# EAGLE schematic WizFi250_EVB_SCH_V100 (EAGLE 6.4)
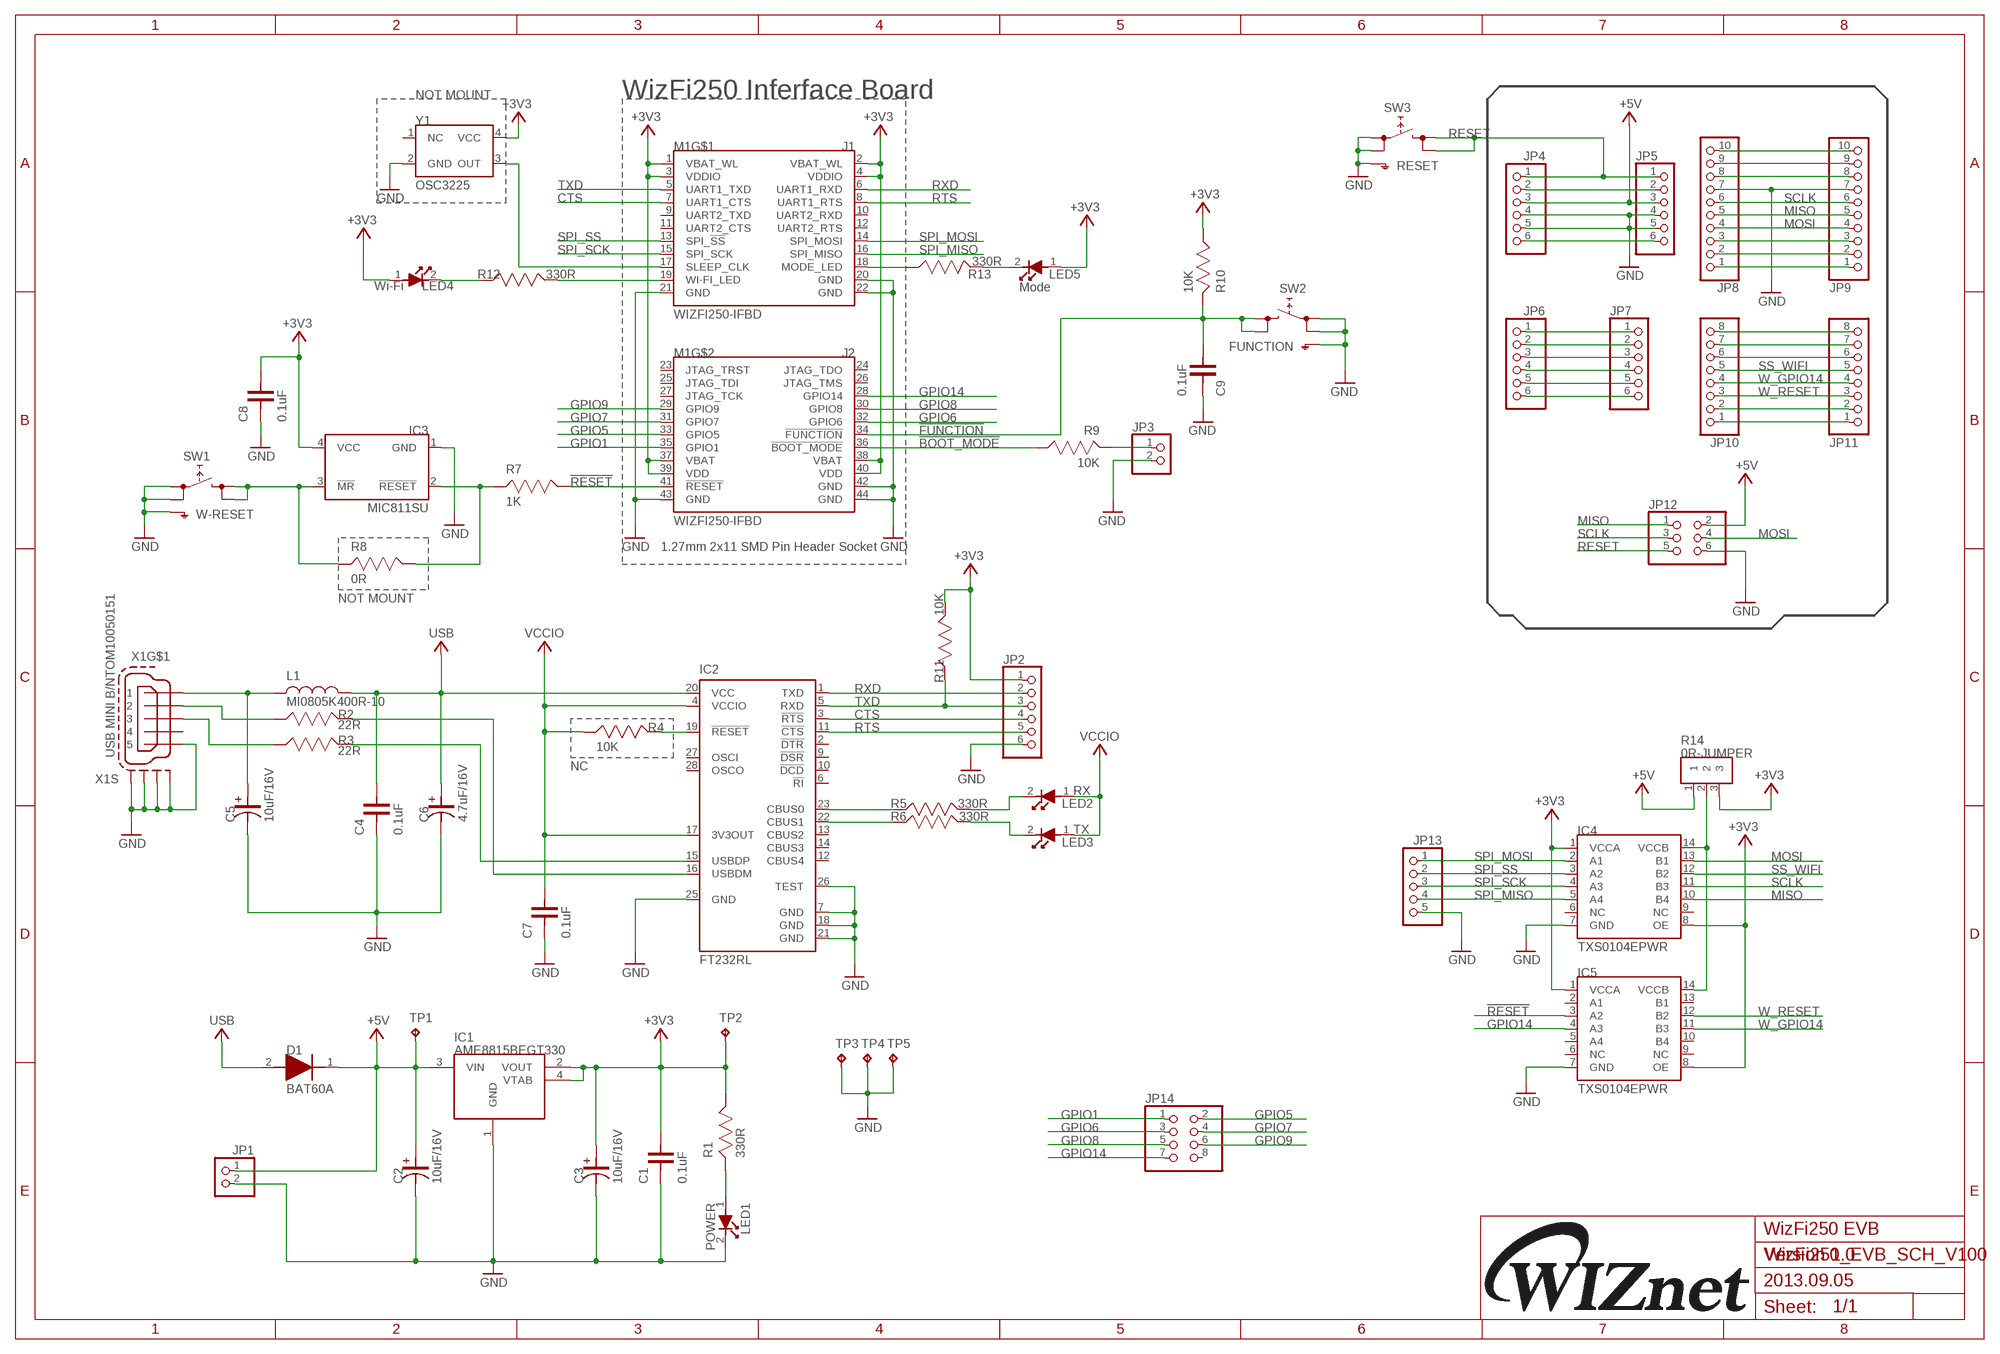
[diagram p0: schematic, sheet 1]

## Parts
C1  0.1uF  C-1608  [C-1608]
C2  10uF/16V  C-3216(TANTAL)  [C-3216(TANTAL)]
C3  10uF/16V  C-3216(TANTAL)  [C-3216(TANTAL)]
C4  0.1uF  C-1608  [C-1608]
C5  10uF/16V  C-3216(TANTAL)  [C-3216(TANTAL)]
C6  4.7uF/16V  C-3216(TANTAL)  [C-3216(TANTAL)]
C7  0.1uF  C-1608  [C-1608]
C8  0.1uF  C-1608  [C-1608]
C9  0.1uF  C-1608  [C-1608]
D1  BAT60A  [BAT60A]
IC1  AME8815BEGT330  [SOT-223]
IC2  FT232RL  [SSOP28]
IC3  MIC811SU  [MIC811SU]
IC4  TXS0104EPWR  [TXS0104EPWR]
IC5  TXS0104EPWR  [TXS0104EPWR]
JP1  PINHD-1X2  [1X02]
JP2  PINHD-1X6  [1X06]
JP3  PINHD-1X2  [1X02]
JP4  PINHD-1X6  [1X06]
JP5  PINHD-1X6  [1X06]
JP6  PINHD-1X6  [1X06]
JP7  PINHD-1X6  [1X06]
JP8  PINHD-1X10  [1X10]
JP9  PINHD-1X10  [1X10]
JP10  PINHD-1X8  [1X08]
JP11  PINHD-1X8  [1X08]
JP12  PINHD-2X3  [2X03]
JP13  PINHD-1X5  [1X05]
JP14  PINHD-2X4  [2X04]
L1  MI0805K400R-10  L-2012  [L-2012]
LED1  POWER  LED-1608  [LED-1608]
LED2  RX  LED-1608  [LED-1608]
LED3  TX  LED-1608  [LED-1608]
LED4  Wi-Fi  LED-1608  [LED-1608]
LED5  Mode  LED-1608  [LED-1608]
M1  WIZFI250-IFBD  [WIZFI250-IFBD]
R1  330R  R-1608  [R-1608]
R2  22R  R-1608  [R-1608]
R3  22R  R-1608  [R-1608]
R4  10K  R-1608  [R-1608]
R5  330R  R-1608  [R-1608]
R6  330R  R-1608  [R-1608]
R7  1K  R-1608  [R-1608]
R8  0R  R-1608  [R-1608]
R9  10K  R-1608  [R-1608]
R10  10K  R-1608  [R-1608]
R11  10K  R-1608  [R-1608]
R12  330R  R-1608  [R-1608]
R13  330R  R-1608  [R-1608]
R14  0R-JUMPER  R-1608-JUMPER  [R-1608-JUMPER]
SW1  W-RESET  SKHMPSE010  [SKHMPXE010]
SW2  FUNCTION  SKHMPSE010  [SKHMPXE010]
SW3  RESET  SKHMPSE010  [SKHMPXE010]
TP1  TPB1,27  [B1,27]
TP2  TPB1,27  [B1,27]
TP3  TPB1,27  [B1,27]
TP4  TPB1,27  [B1,27]
TP5  TPB1,27  [B1,27]
X1  USB MINI B/NTOM10050151  MINI-USB-SCHIELD-32005-201  [32005-201]
Y1  OSC3225  [OSC3225]

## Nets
!BOOT_MODE: M1.36(!BOOT_MODE) R9.2
!FUNCTION: C9.2 M1.34(!FUNCTION) R10.1 SW2.3(2.1) SW2.4(2.2)
!RESET: IC5.3(A2) M1.41(!RESET) R7.2
+3V3: C1.2 C3.1 C8.2 IC1.2(VOUT) IC1.4(VTAB) IC3.4(VCC) IC4.1(VCCA) IC4.8(OE) IC5.1(VCCA) IC5.8(OE) JP2.1 LED4.1 LED5.1 M1.1(VBAT_WL) M1.2(VBAT_WL) M1.3(VDDIO) M1.4(VDDIO) M1.37(VBAT) M1.38(VBAT) M1.39(VDD) M1.40(VDD) R1.2 R10.2 R11.2 R14.3 TP2.TP Y1.4(VCC)
+5V: C2.1 D1.1 IC1.3(VIN) JP1.1 JP4.3 JP5.3 JP12.2 R14.1 TP1.TP
CTS: IC2.3(!RTS) JP2.4 M1.7(UART1_CTS)
GND: C1.1 C2.2 C3.2 C4.1 C5.2 C6.2 C7.1 C8.1 C9.1 IC1.1(GND) IC2.7(GND) IC2.18(GND) IC2.21(GND) IC2.25(GND) IC2.26(TEST) IC3.1(GND) IC4.7(GND) IC5.7(GND) JP1.2 JP2.6 JP3.2 JP4.4 JP4.5 JP5.4 JP5.5 JP8.7 JP9.7 JP12.6 JP13.5 LED1.2 M1.20(GND) M1.21(GND) M1.22(GND) M1.42(GND) M1.43(GND) M1.44(GND) SW1.1(1.1) SW1.2(1.2) SW1.5(SH) SW2.1(1.1) SW2.2(1.2) SW2.5(SH) SW3.1(1.1) SW3.2(1.2) SW3.5(SH) TP3.TP TP4.TP TP5.TP X1.5 X1.M1(S:S1) X1.M2(S:S2) X1.M3(S:S3) X1.M4(S:S4) Y1.2(GND)
GPIO1: JP14.1 M1.35(GPIO1)
GPIO5: JP14.2 M1.33(GPIO5)
GPIO6: JP14.3 M1.32(GPIO6)
GPIO7: JP14.4 M1.31(GPIO7)
GPIO8: JP14.5 M1.30(GPIO8)
GPIO9: JP14.6 M1.29(GPIO9)
GPIO14: IC5.4(A3) JP14.7 M1.28(GPIO14)
MISO: IC4.10(B4) JP8.5 JP9.5 JP12.1
MOSI: IC4.13(B1) JP8.4 JP9.4 JP12.4
N$1: IC4.14(VCCB) IC5.14(VCCB) R14.2
N$2: R2.1 X1.2
N$3: R3.1 X1.3
N$4: LED1.1 R1.1
N$5: JP3.1 R9.1
N$6: IC2.16(USBDM) R2.2
N$7: IC2.15(USBDP) R3.2
N$8: IC2.19(!RESET) R4.2
N$9: IC3.2(!RESET) R7.1 R8.2
N$16: LED2.2 R5.2
N$17: LED3.2 R6.2
N$18: JP4.2 JP5.2
N$22: JP4.6 JP5.6
N$23: JP6.1 JP7.1
N$24: JP6.2 JP7.2
N$25: JP6.3 JP7.3
N$26: JP6.4 JP7.4
N$27: JP6.5 JP7.5
N$28: JP6.6 JP7.6
N$29: JP8.10 JP9.10
N$30: JP8.9 JP9.9
N$31: JP8.8 JP9.8
N$36: JP8.3 JP9.3
N$37: JP8.2 JP9.2
N$38: JP8.1 JP9.1
N$39: JP10.8 JP11.8
N$40: JP10.7 JP11.7
N$41: JP10.6 JP11.6
N$45: JP10.2 JP11.2
N$46: JP10.1 JP11.1
N$50: M1.17(SLEEP_CLK) Y1.3(OUT)
N$51: M1.19(WI-FI_LED) R12.2
N$52: LED4.2 R12.1
N$64: M1.18(MODE_LED) R13.1
N$65: LED5.2 R13.2
RESET: JP4.1 JP5.1 JP12.5 SW3.3(2.1) SW3.4(2.2)
RTS: IC2.11(!CTS) JP2.5 M1.8(UART1_RTS)
RX-LED: IC2.23(CBUS0) R5.1
RXD: IC2.1(TXD) JP2.2 M1.6(UART1_RXD)
SCLK: IC4.11(B3) JP8.6 JP9.6 JP12.3
SPI_MISO: IC4.5(A4) JP13.4 M1.16(SPI_MISO)
SPI_MOSI: IC4.2(A1) JP13.1 M1.14(SPI_MOSI)
SPI_SCK: IC4.4(A3) JP13.3 M1.15(SPI_SCK)
SPI_SS: IC4.3(A2) JP13.2 M1.13(SPI_!SS)
SS_WIFI: IC4.12(B2) JP10.5 JP11.5
TX-LED: IC2.22(CBUS1) R6.1
TXD: IC2.5(RXD) JP2.3 M1.5(UART1_TXD) R11.1
USB: C4.2 C6.1 D1.2 IC2.20(VCC) L1.2
VCC: C5.1 L1.1 X1.1
VCCIO: C7.2 IC2.4(VCCIO) IC2.17(3V3OUT) LED2.1 LED3.1 R4.1
W_GPIO14: IC5.11(B3) JP10.4 JP11.4
W_RESET: IC5.12(B2) JP10.3 JP11.3
WI-FI_RST: IC3.3(!MR) R8.1 SW1.3(2.1) SW1.4(2.2)
Unconnected: IC2.2(!DTR) IC2.6(!RI) IC2.9(!DSR) IC2.10(!DCD) IC2.12(CBUS4) IC2.13(CBUS2) IC2.14(CBUS3) IC2.27(OSCI) IC2.28(OSCO) IC4.6(NC) IC4.9(NC) IC5.2(A1) IC5.5(A4) IC5.6(NC) IC5.9(NC) IC5.10(B4) IC5.13(B1) JP14.8 M1.9(UART2_TXD) M1.10(UART2_RXD) M1.11(UART2_CTS) M1.12(UART2_RTS) M1.23(JTAG_TRST) M1.24(JTAG_TDO) M1.25(JTAG_TDI) M1.26(JTAG_TMS) M1.27(JTAG_TCK) X1.4 Y1.1(NC)

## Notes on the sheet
- NOT MOUNT | WizFi250 Inferface Board
- J1
- J2
- 1.27mm 2x11 SMD Pin Header Socket
- NOT MOUNT
- NC
- WizFi250 EVB
- Version 1.0
- 2013.09.05

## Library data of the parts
C1 C4 C7-C9 = CAP:C-1608
C2 C3 C5 C6 = CAP:C-3216(TANTAL)
D1 = DIODE:BAT60A
IC1 = RECULATOR:AME8815BEGT330
IC2 = ftdichip:FT232R: Source: http://www.ftdichip.com/Documents/DataSheets/DS_FT232R_v104.pdf; MPN: FT232RL; OC_FARNELL: 1146032; OC_NEWARK: 91K9918
IC3 = IC:MIC811SU
IC4 IC5 = IC:TXS0104EPWR
JP1 JP3 = pinhead:PINHD-1X2: PIN HEADER
JP2 JP4-JP7 = pinhead:PINHD-1X6: PIN HEADER
JP8 JP9 = pinhead:PINHD-1X10: PIN HEADER
JP10 JP11 = pinhead:PINHD-1X8: PIN HEADER
JP12 = pinhead:PINHD-2X3: PIN HEADER
JP13 = pinhead:PINHD-1X5: PIN HEADER
JP14 = pinhead:PINHD-2X4: PIN HEADER
L1 = INDUCTOR:L-2012
LED1-LED5 = DIODE:LED-1608
M1 = WIZnet:WIZFI250-IFBD
R1-R13 = RESISTOR:R-1608
R14 = RESISTOR:R-1608-JUMPER
SW1-SW3 = switch:SKHMP*E010: 6.2 X 6.5mm TACT Switch (SMD) Source: http://www3.alps.co.jp/WebObjects/catalog.woa/PDF/E/Switch/Tact/SKHM/SKHM.PDF
TP1-TP5 = testpad:TP: Test pad
X1 = USB:MINI-USB-SCHIELD-: MINI USB-B Conector Source: www.cypressindustries.com; OC_FARNELL: unknown; OC_NEWARK: unknown
Y1 = X-TAL:OSC3225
